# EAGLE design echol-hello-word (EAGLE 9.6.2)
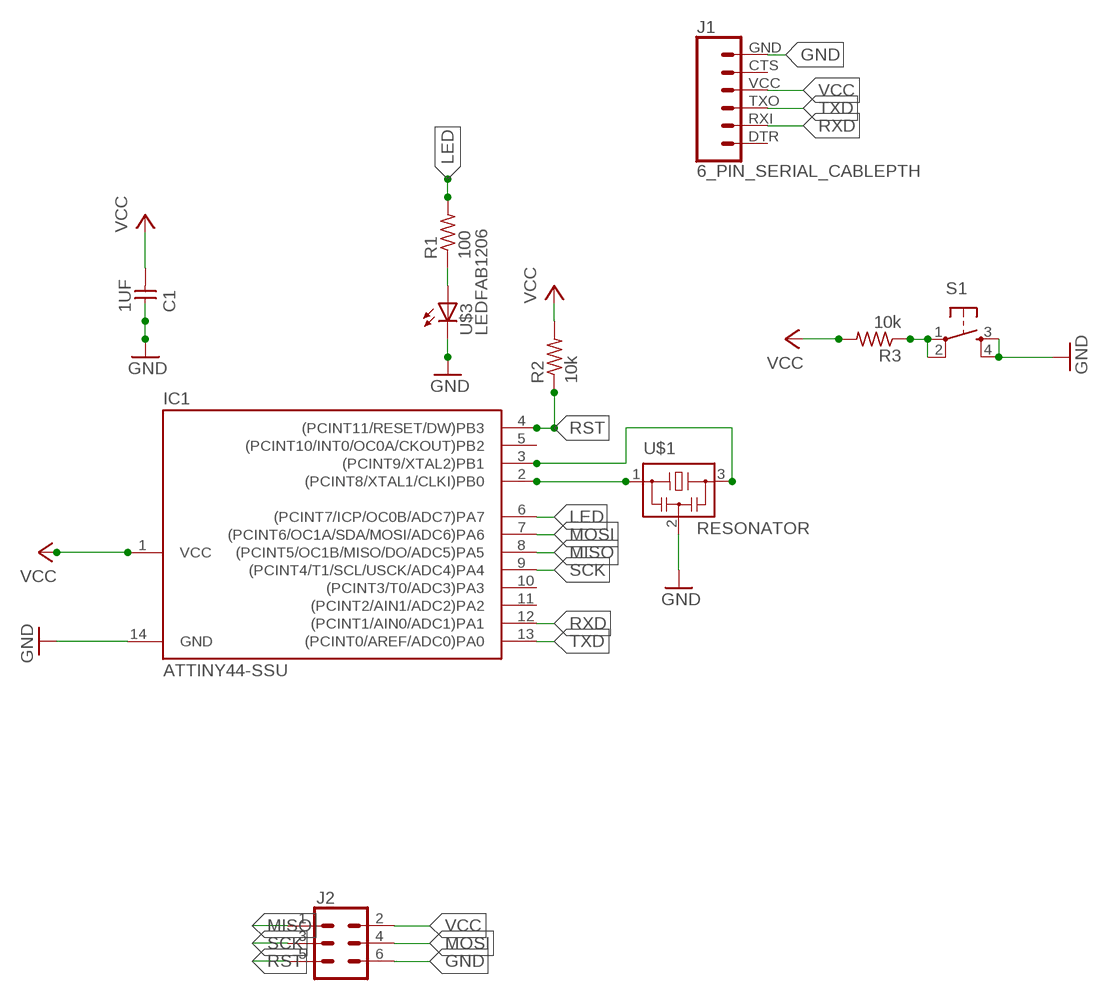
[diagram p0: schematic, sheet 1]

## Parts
C1  1UF  CAP-UNPOLARIZEDFAB  [C1206FAB]
IC1  ATTINY44-SSU  [SOIC14]
J1  6_PIN_SERIAL_CABLEPTH  [FTDI_BASIC]
J2  CONN_03X22X3_SILK_MALE_PTH  [2X3]
R1  100  RES-US1206FAB  [R1206FAB]
R2  10k  RES-US1206FAB  [R1206FAB]
R3  10k  RES-US1206FAB  [R1206FAB]
S1  6MM_SWITCH6MM_SWITCH  [6MM_SWITCH]
U$1  RESONATOR  [EFOBM]
U$3  LEDFAB1206  [LED1206FAB]

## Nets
GND: C1.1 IC1.14(GND) J1.GND J2.6 S1.3(S) S1.4(S1) U$1.2 U$3.2(C)
LED: IC1.6((PCINT7/ICP/OC0B/ADC7)PA7) R1.2
MISO: IC1.8((PCINT5/OC1B/MISO/DO/ADC5)PA5) J2.1
MOSI: IC1.7((PCINT6/OC1A/SDA/MOSI/ADC6)PA6) J2.4
N$1: R1.1 U$3.1(A)
N$2: IC1.2((PCINT8/XTAL1/CLKI)PB0) U$1.1
N$3: IC1.3((PCINT9/XTAL2)PB1) U$1.3
N$5: R3.1 S1.1(P) S1.2(P1)
RST: IC1.4((PCINT11/RESET/DW)PB3) J2.5 R2.1
RXD: IC1.12((PCINT1/AIN0/ADC1)PA1) J1.RXI
SCK: IC1.9((PCINT4/T1/SCL/USCK/ADC4)PA4) J2.3
TXD: IC1.13((PCINT0/AREF/ADC0)PA0) J1.TXO
VCC: C1.2 IC1.1(VCC) J1.VCC J2.2 R2.2 R3.2
Unconnected: IC1.5((PCINT10/INT0/OC0A/CKOUT)PB2) IC1.10((PCINT3/T0/ADC3)PA3) IC1.11((PCINT2/AIN1/ADC2)PA2) J1.CTS J1.DTR

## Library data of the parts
C1 = fab:CAP-UNPOLARIZED
IC1 = fab:ATTINY44
J1 = SparkFun-Connectors:6_PIN_SERIAL_CABLE: 6-pin header connection for use with the "FTDI BASIC" pinout - CABLE SIDE. Also known as "Arduino Serial Program Header". This is used on a design to provide a 6-pin connection point for serial communication usually from a USB cable (D+/D-) to these headers (RX/TX). It also has the remaining pins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
J2 = SparkFun-Connectors:CONN_03X2: Multi connection point. Often used as Generic Header-pin footprint for 0.1 inch spaced/style header connections You can populate with any combo of single row headers, but if you'd like an exact match, check these: Header - 2x3 (Male, 0.1") (PRT-12807) Header - 2x3 (Female, 0.1") (PRT-13010) 2x3 Pin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; PROD_ID: CONN-09701
R1-R3 = fab:RES-US: Resistor (US Symbol)
S1 = fab:6MM_SWITCH: OMRON SWITCH
U$1 = fab:RESONATOR
U$3 = fab:LED: LED

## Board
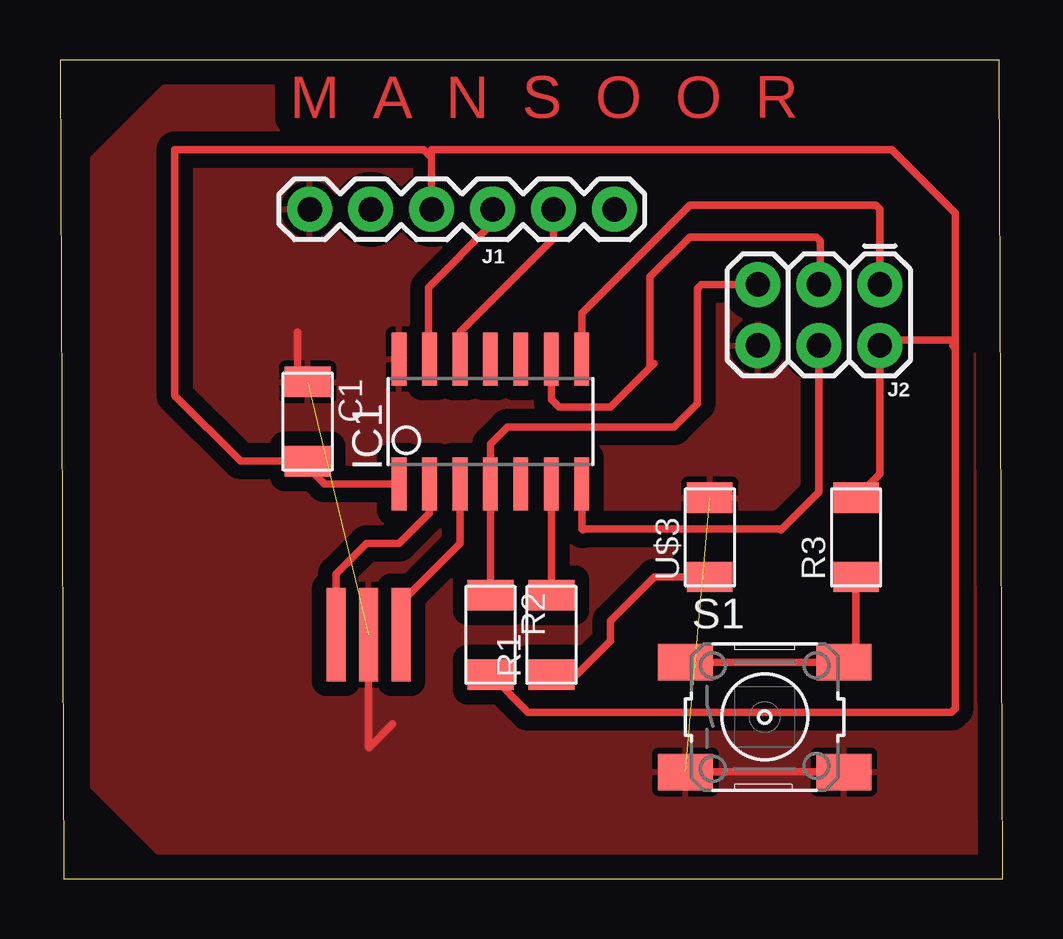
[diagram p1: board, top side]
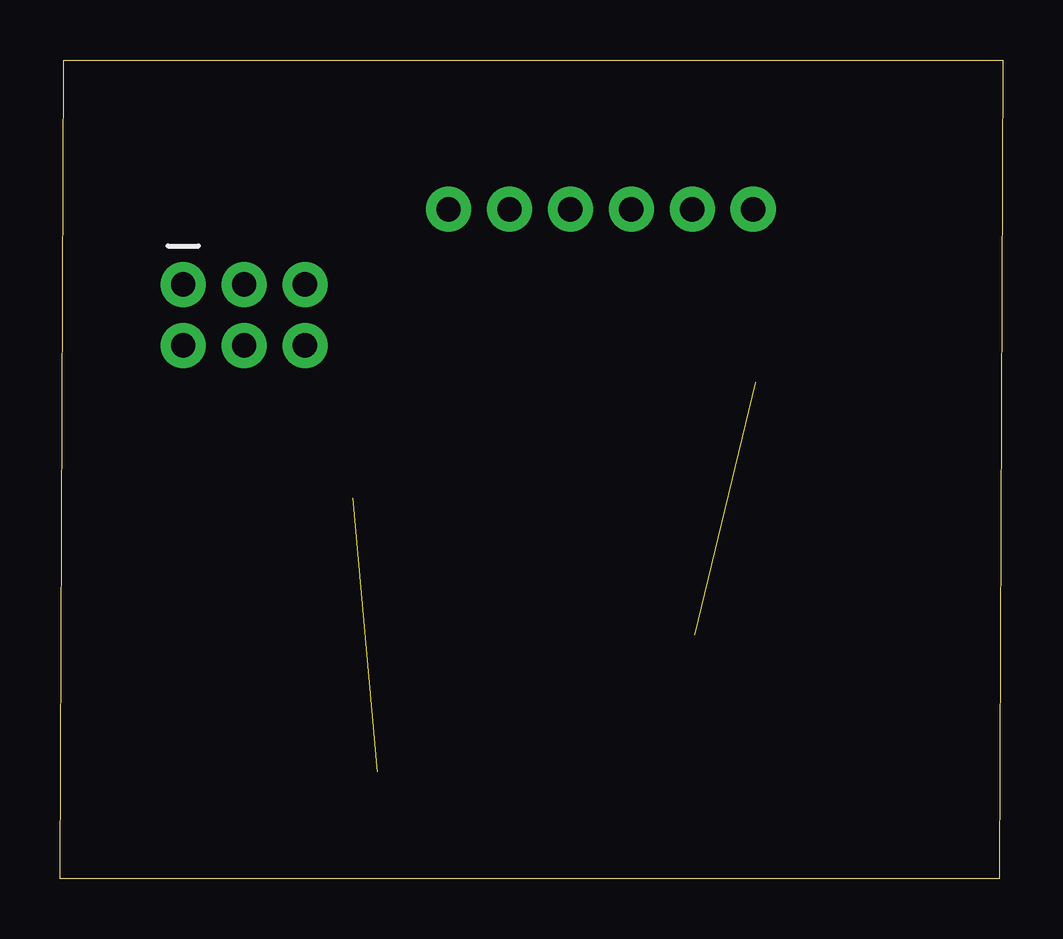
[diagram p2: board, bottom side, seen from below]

Size 39.31 x 34.13 mm. Coordinates in mm from the lower left corner, seen from the top.
Outline: 0.17,0 39.31,0 39.15,34.12 0,34.12 0.17,0
Copper layers (1*16): Top 0.035mm / dielectric 1.5mm / Bottom 0.035mm
Design rules "default": minimum track width 10mil, minimum drill 24mil, track to track 8mil, track to pad 8mil, pad to pad 8mil, via to via 8mil, smd to smd 8mil, copper to edge 40mil, drill to drill 8mil, minimum pad ring 10mil, minimum via ring 8mil, stop-mask expansion 4mil, vias tented up to drill 0mil, thermal gap 10mil

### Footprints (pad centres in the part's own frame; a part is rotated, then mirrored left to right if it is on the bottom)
C1206FAB = smd 1.27 x 1.905: 1 -1.651,0; 2 1.651,0
SOIC14 = smd 0.61 x 2.21: 1 -3.81,-2.603; 2 -2.54,-2.603; 3 -1.27,-2.603; 4 0,-2.603; 5 1.27,-2.603; 6 2.54,-2.603; 7 3.81,-2.603; 8 3.81,2.603; 9 2.54,2.603; 10 1.27,2.603; 11 0,2.603; 12 -1.27,2.603; 13 -2.54,2.603; 14 -3.81,2.603
FTDI_BASIC = drill 1.016 pad 1.88: CTS 10.16,0; DTR 0,0; GND 12.7,0; RXI 2.54,0; TXO 5.08,0; VCC 7.62,0
2X3 = drill 1.016 pad 1.88: 1 0,0; 2 0,2.54; 3 2.54,0; 4 2.54,2.54; 5 5.08,0; 6 5.08,2.54
R1206FAB = smd 1.27 x 1.905: 1 -1.651,0; 2 1.651,0
6MM_SWITCH = smd 2.286 x 1.524: 1 -3.302,2.286; 2 3.302,2.286; 3 -3.302,-2.286; 4 3.302,-2.286
EFOBM = smd 0.8 x 3.9: 1 -1.35,0; 2 0,0; 3 1.35,0
LED1206FAB = smd 1.27 x 1.905: 1 -1.651,0; 2 1.651,0

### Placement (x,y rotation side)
C1  10.33,19.05 270 top
IC1  17.95,19.05 0 top
J1  23.11,27.9 180 top
J2  34.18,24.77 180 top
R1  20.49,10.16 90 top
R2  17.95,10.16 270 top
R3  33.19,14.22 90 top
S1  29.38,6.73 0 top
U$1  12.87,10.16 0 top
U$3  27.09,14.22 90 top

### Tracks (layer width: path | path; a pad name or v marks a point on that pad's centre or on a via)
GND  (2 unrouted)
  Top 0.305: S1.3 S1.4 | C1.1 9.91,21.12 9.91,22.78 | U$1.2 12.87,5.46 12.88,5.45 13.87,6.44
  pour Top (isolate 0.61): 1.32,3.8 4.29,0.83 38.3,0.83 38.3,29.55 33.85,34.01 5.28,34.01 1.32,30.05
LED
  Top 0.305: R1.2 IC1.6
MISO
  Top 0.305: 21.76,21.63 IC1.8 21.76,23.57 26.25,28.07 27.08,28.07 27.24,28.07 34.01,28.07 34.18,27.9 J2.1
MOSI
  Top 0.305: IC1.7 21.76,14.57 | 21.79,14.53 21.76,14.57 | 21.76,14.57 30.01,14.57 30.05,14.53 31.64,16.12 J2.4
N$1
  Top 0.305: U$3.1 24.79,12.57 22.95,10.73 22.95,9.91 21.55,8.51 R1.1
N$2
  Top 0.305: IC1.2 15.41,15.24 14.14,13.97 12.79,13.97 11.52,12.7 U$1.1
N$3
  Top 0.305: U$1.3 14.22,11.51 16.68,13.97 IC1.3
N$5
  Top 0.305: S1.1 S1.2 33.19,9.53 R3.1
RST
  Top 0.305: R2.1 IC1.4 17.95,18.11 18.66,18.82 25.59,18.82 26.58,19.81 26.58,24.6 26.75,24.77 J2.5 28.56,24.77
RXD
  Top 0.305: J1.RXI 20.57,26.68 16.68,22.78 IC1.12
SCK
  Top 0.305: J2.3 31.7,24.83 31.7,26.58 31.53,26.75 26.25,26.75 24.6,25.09 24.6,21.3 | IC1.9 20.49,19.96 20.8,19.65 22.95,19.65 24.6,21.3 | 24.6,21.3 24.77,21.46
TXD
  Top 0.254: 15.35,21.65 IC1.13
  Top 0.305: J1.TXO 18.03,27.32 15.35,24.64 15.35,21.65
VCC
  Top 0.305: 33.19,15.68 R3.2 34.18,16.87 J2.2 34.4,22.45 37.31,22.45 | 37.31,22.12 37.31,22.45 | 37.31,22.45 37.31,27.74 34.67,30.38 15.49,30.38 15.49,30.05 | 18,8.46 R2.2 19.52,6.93 37.15,6.93 37.31,7.1 37.31,22.12 | J1.VCC 15.49,30.05 | 37.21,22.23 37.31,22.12 | 10.51,17.21 C1.2 10.07,17.4 | 10.07,17.4 7.53,17.4 4.79,20.14 4.79,30.38 15.16,30.38 15.49,30.05 | IC1.1 11.02,16.45 10.07,17.4

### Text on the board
Top: M A N S O O R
